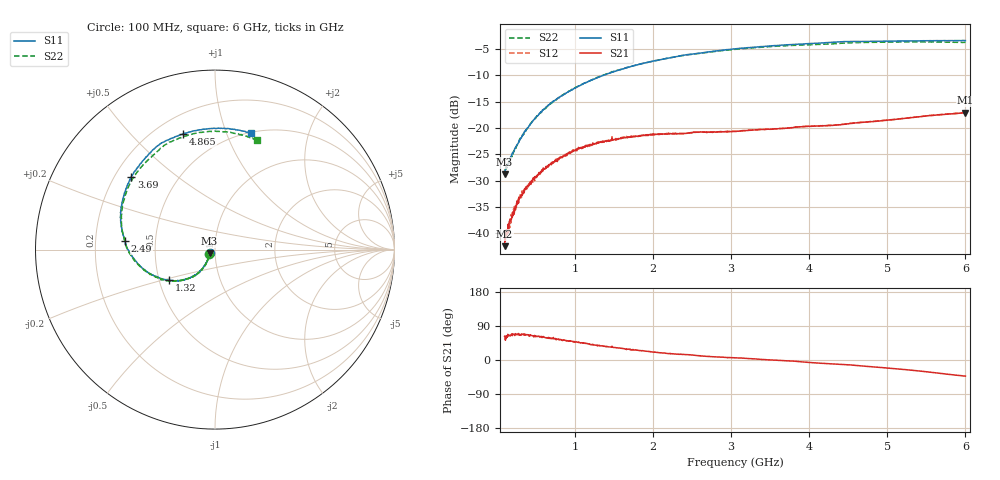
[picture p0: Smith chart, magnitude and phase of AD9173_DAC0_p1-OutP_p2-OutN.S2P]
! Created Thu Dec 01 14:57:47 2016
# mhz S ma R 50
! 2 Port Network Data from Sweep1.SP1.SP block
! freq  magS11  angS11  magS21  angS21  magS12  angS12  magS22  angS22
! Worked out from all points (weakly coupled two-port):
!   1181 points, 100 MHz to 6 GHz, reference 50 ohm
!   highest |S21| = -17.07 dB at 6 GHz (marker M1); lowest = -42.5 dB at 100 MHz (marker M2)
!   lowest |S11| = -28.8 dB at 100 MHz (marker M3), VSWR 1.08, Z = 47 - j1.86 ohm
!   |S11| at or under -10 dB: start of sweep to 1.363 GHz
!   |S22| runs from -28.1 to -3.6 dB; largest |S21 - S12| = 0.0055
!   S11 on the Smith chart (normalised r, x): 100 MHz: 0.94, -0.04; 1.32 GHz: 0.56, -0.21; 2.49 GHz: 0.33, +0.04; 3.69 GHz: 0.27, +0.35; 4.865 GHz: 0.31, +0.72; 6 GHz: 0.51, +1.22
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100  0.03637 -147.0  0.007506 62.7  0.008363 67.2  0.03939 -143.6
145  0.04526 -135.1  0.01214 66.8  0.01046 67.8  0.04452 -134.0
210  0.05793 -127.9  0.01474 68.1  0.01605 68.8  0.05845 -126.4
270  0.07047 -125.5  0.01959 68.1  0.01977 67.0  0.07151 -125.0
300  0.07736 -124.8  0.02189 65.3  0.02318 69.4  0.0789 -123.4
380  0.09713 -122.4  0.02664 66.6  0.02732 70.3  0.09692 -122.4
445  0.1124 -123.3  0.03161 65.1  0.03197 65.0  0.1133 -122.4
700  0.1747 -126.7  0.04541 57.8  0.04521 56.7  0.172 -126.8
875  0.2109 -132.0  0.05426 51.4  0.05589 52.2  0.2139 -131.9
1085  0.2585 -138.0  0.06506 45.7  0.0638 43.9  0.2596 -138.4
1320  0.3075 -146.2  0.0732 37.4  0.07225 38.4  0.3086 -145.7
1690  0.3804 -158.4  0.08229 28.4  0.08201 28.5  0.3795 -158.0
2070  0.4426 -171.0  0.08713 19.3  0.08695 19.8  0.4437 -170.5
2490  0.5023 174.7  0.08983 13.4  0.08984 13.1  0.5022 175.4
3050  0.5653 158.1  0.09291 5.8  0.09303 5.6  0.561 158.1
3690  0.6184 139.0  0.09939 -1.7  0.09974 -2.0  0.605 138.8
4035  0.6374 129.3  0.104 -7.1  0.104 -6.7  0.6203 128.7
4460  0.6645 116.9  0.1086 -12.0  0.109 -11.9  0.6437 116.7
4865  0.6683 105.2  0.1162 -19.0  0.1166 -18.8  0.6536 104.3
5020  0.6713 100.9  0.1193 -21.6  0.1195 -21.4  0.6573 99.7
5500  0.6763 87.2  0.1304 -30.9  0.1301 -31.1  0.659 84.7
6000  0.6786 72.9  0.1402 -42.7  0.1405 -42.6  0.6532 68.8
